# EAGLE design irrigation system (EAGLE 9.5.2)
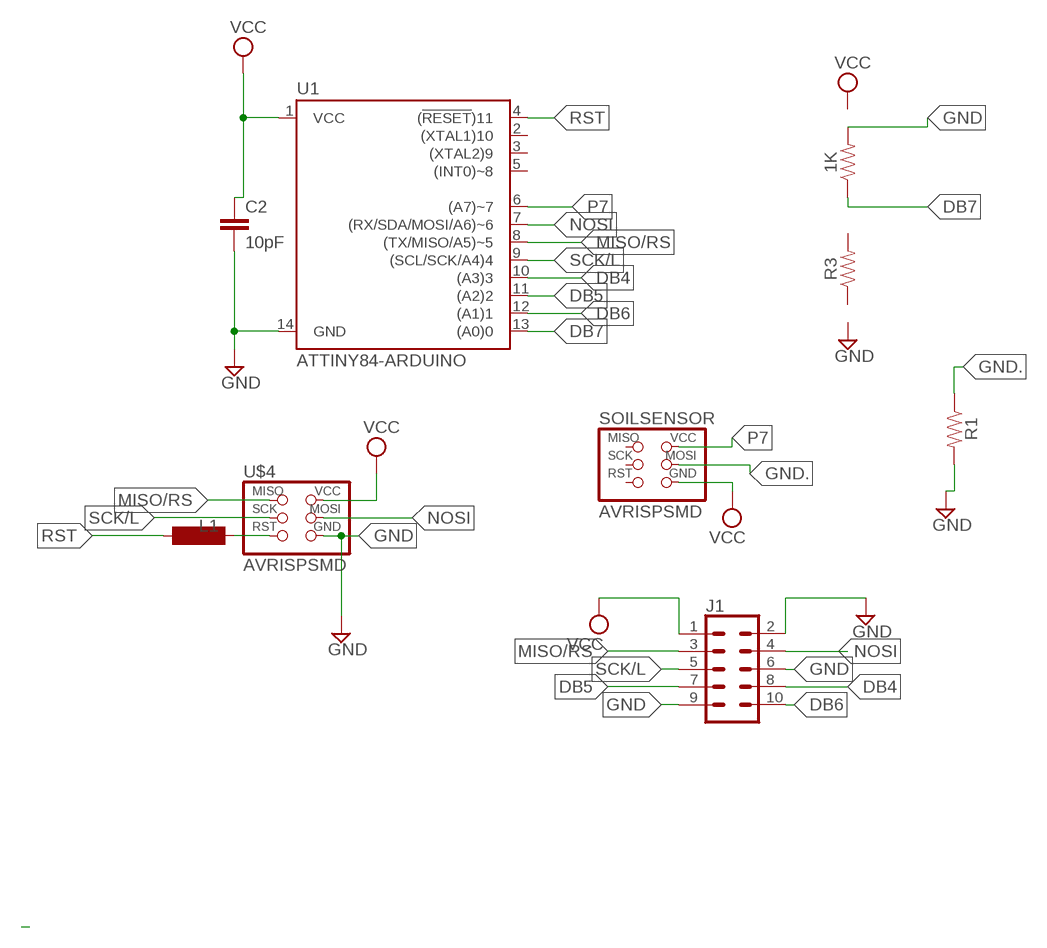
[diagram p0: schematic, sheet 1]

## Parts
1K  RESISTOR1206  [1206]
C2  10pF  10PF-0603-50V-5%  [0603]
J1  CONN_05X2SHD_SMD  [2X5-SHROUDED_SMD]
L1  SM-1206  [SM-1206]
R1  RESISTOR1206  [1206]
R3  RESISTOR1206  [1206]
SOILSENSOR  AVRISPSMD  [2X03SMD]
U1  ATTINY84-ARDUINO  [SO14]
U$4  AVRISPSMD  [2X03SMD]

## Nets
DB4: J1.8 U1.10((A3)3)
DB5: J1.7 U1.11((A2)2)
DB6: J1.10 U1.12((A1)1)
DB7: 1K.1 U1.13((A0)0)
GND: 1K.2 C2.2 J1.2 J1.6 J1.9 R1.2 U1.14(GND) U$4.6(GND)
GND.: R1.1 SOILSENSOR.4(MOSI)
MISO/RS: J1.3 U1.8((TX/MISO/A5)~5) U$4.1(MISO)
N$6: L1.2 U$4.5(RST)
NOSI: J1.4 U1.7((RX/SDA/MOSI/A6)~6) U$4.4(MOSI)
P7: SOILSENSOR.2(VCC) U1.6((A7)~7)
RST: L1.1 U1.4((!RESET!)11)
SCK/L: J1.5 U1.9((SCL/SCK/A4)4) U$4.3(SCK)
VCC: C2.1 J1.1 SOILSENSOR.6(GND) U1.1(VCC) U$4.2(VCC)
Unconnected: R3.1 R3.2 SOILSENSOR.1(MISO) SOILSENSOR.3(SCK) SOILSENSOR.5(RST) U1.2((XTAL1)10) U1.3((XTAL2)9) U1.5((INT0)~8)

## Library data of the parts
1K R1 R3 = SparkFun-Resistors:RESISTOR: Generic Resistor Package
C2 = SparkFun-Capacitors:10PF: 10pF ceramic capacitors; PROD_ID: CAP-11812
J1 = SparkFun-Connectors:CONN_05X2: Multi connection point. Often used as Generic Header-pin footprint for 0.1 inch spaced/style header connections For AVR SPI programming port, see special device with nice symbol: "AVR_SPI_PROG_5x2.dev" You can populate with any combo of single row headers, but if you'd like an exact match, check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; PROD_ID: CONN-09508
L1 = inductor-neosid:SM-1206: INDUCTOR; OC_FARNELL: unknown; OC_NEWARK: unknown
SOILSENSOR U$4 = fab:AVRISP
U1 = SparkFun-IC-Microcontroller:ATTINY84-ARDUINO; PROD_ID: IC-14155

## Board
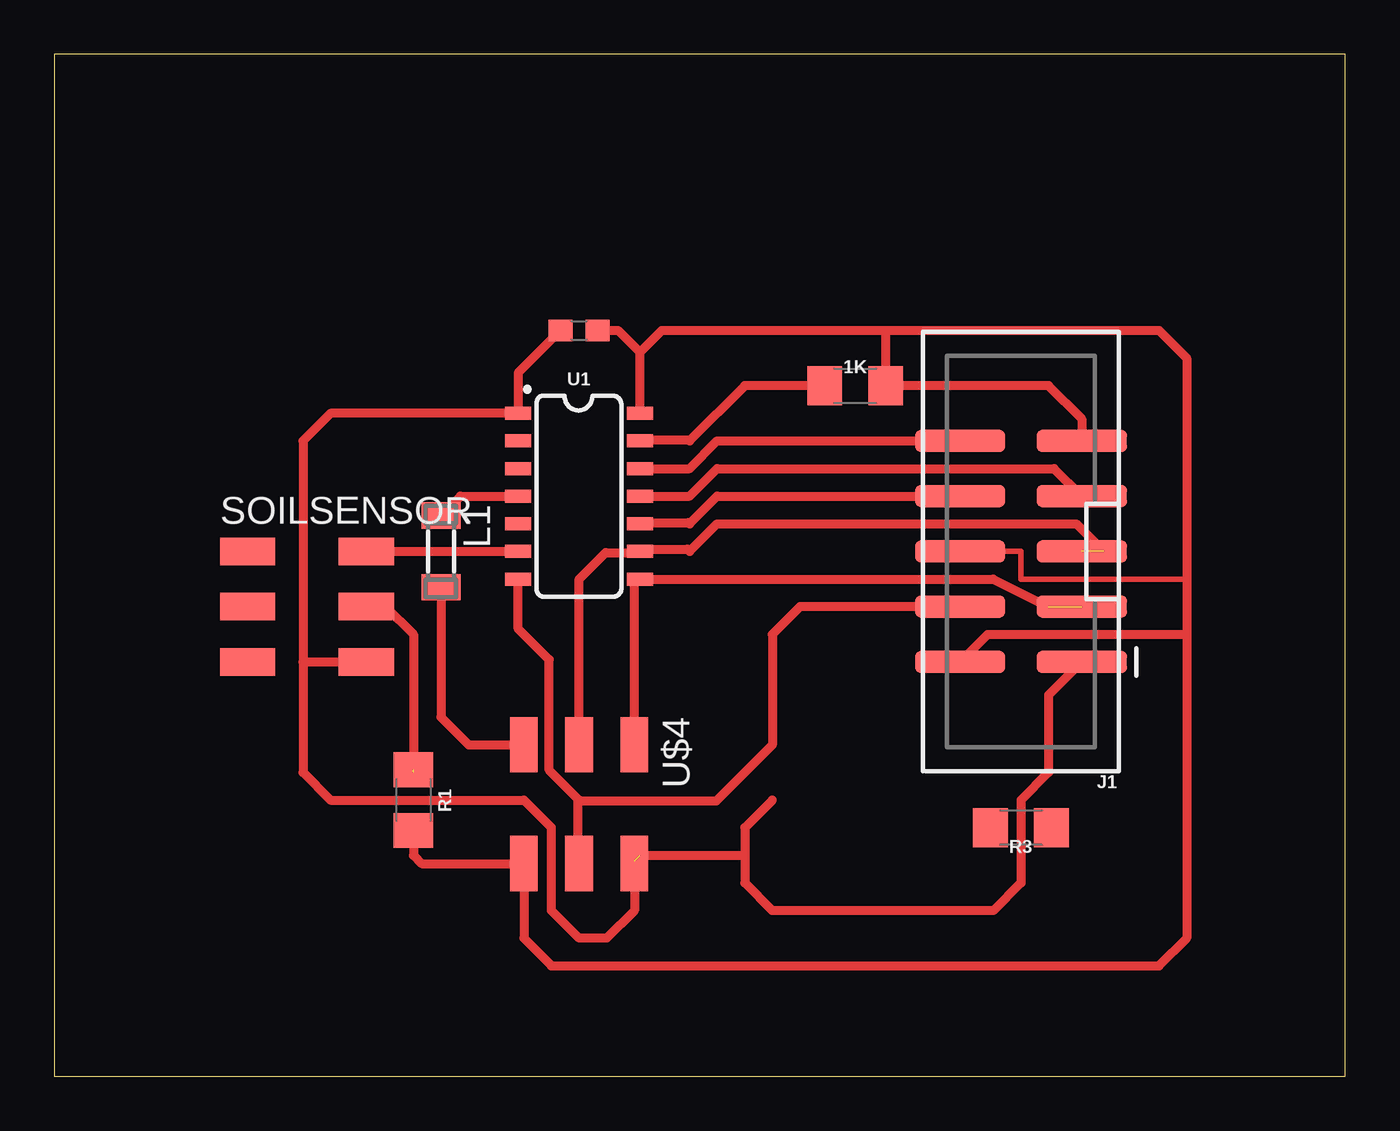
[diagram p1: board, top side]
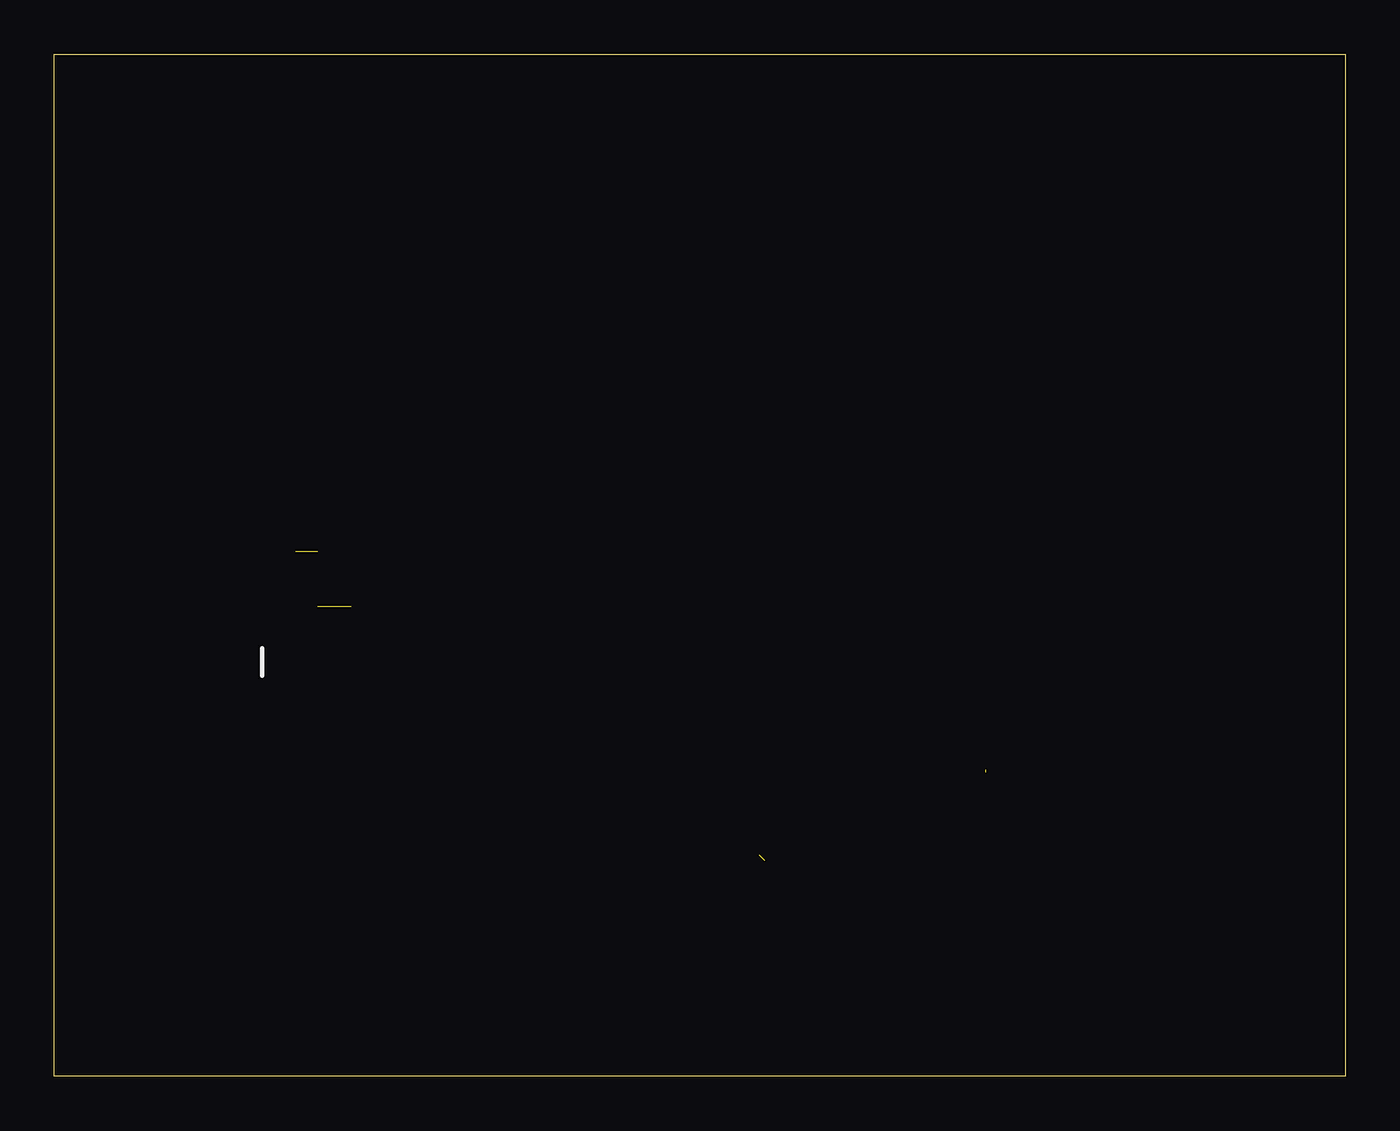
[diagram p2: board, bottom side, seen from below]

Size 59.36 x 46.98 mm. Coordinates in mm from the lower left corner, seen from the top.
Outline: 0,0 59.36,0 59.36,46.98 0,46.98 0,0
Copper layers (1*16): Top 0.035mm / dielectric 1.5mm / Bottom 0.035mm
Design rules "default": minimum track width 6mil, minimum drill 0.35mm, track to track 6mil, track to pad 6mil, pad to pad 6mil, via to via 6mil, smd to smd 6mil, copper to edge 40mil, drill to drill 6mil, minimum pad ring 10mil, minimum via ring 8mil, stop-mask expansion 4mil, vias tented up to drill 0mil, thermal gap 10mil

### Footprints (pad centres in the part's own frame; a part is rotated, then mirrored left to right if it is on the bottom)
1206 = smd 1.6 x 1.8: 1 -1.4,0; 2 1.4,0
0603 = smd 1.1 x 1: 1 -0.85,0; 2 0.85,0
2X5-SHROUDED_SMD = smd 4.15 x 1: 1 -2.794,5.08; 2 2.794,5.08; 3 -2.794,2.54; 4 2.794,2.54; 5 -2.794,0; 6 2.794,0; 7 -2.794,-2.54; 8 2.794,-2.54; 9 -2.794,-5.08; 10 2.794,-5.08
SM-1206 = smd 1.2 x 1.8: 1 -1.65,0; 2 1.65,0
2X03SMD = smd 2.54 x 1.27: 1 -2.54,2.54; 2 2.92,2.54; 3 -2.54,0; 4 2.92,0; 5 -2.54,-2.54; 6 2.92,-2.54
SO14 = smd 0.6 x 1.2: 1 -3.81,-2.8; 2 -2.54,-2.8; 3 -1.27,-2.8; 4 0,-2.8; 5 1.27,-2.8; 6 2.54,-2.8; 7 3.81,-2.8; 8 3.81,2.8; 9 2.54,2.8; 10 1.27,2.8; 11 0,2.8; 12 -1.27,2.8; 13 -2.54,2.8; 14 -3.81,2.8

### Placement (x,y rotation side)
1K  36.83,31.75 0 top
C2  24.13,34.29 0 top
J1  44.45,24.13 180 top
L1  17.78,24.13 270 top
R1  16.51,12.7 270 top
R3  44.45,11.43 180 top
SOILSENSOR  11.43,21.59 0 top
U1  24.13,26.67 270 top
U$4  24.13,12.7 270 top

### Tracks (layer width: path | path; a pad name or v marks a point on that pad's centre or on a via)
DB4
  Top 0.152: 26.98,25.3 U1.10 26.98,25.45 | 29.16,25.45 29.21,25.4
  Top 0.406: 26.98,25.45 29.16,25.45 | 29.21,25.4 30.48,26.67 J1.8
DB5
  Top 0.406: U1.11 29.21,26.67 30.48,27.94 45.97,27.94 J1.7
DB6
  Top 0.152: U1.12 26.98,28.04
  Top 0.406: J1.10 30.48,29.21 29.21,27.94 U1.12
DB7
  Top 0.152: U1.13 26.98,29.26 | 29.21,29.21 29.16,29.26
  Top 0.406: 26.98,29.26 29.16,29.26 | 1K.1 31.75,31.75 29.21,29.21
GND
  Top 0.152: C2.2 24.84,34.29 | U1.14 26.52,30.48 | U$4.6 21.64,9.75 | 41.76,24.13 J1.6
  Top 0.254: J1.6 44.45,24.13 44.45,22.86 52.07,22.86
  Top 0.406: U1.14 26.93,33.28 | 26.93,33.28 27.94,34.29 38.1,34.29 | 38.1,34.29 50.8,34.29 52.07,33.02 52.07,22.86 52.07,20.32 | 52.07,20.32 52.07,6.35 50.8,5.08 22.86,5.08 21.59,6.35 U$4.6 16.89,9.78 16.51,10.16 R1.2 | C2.2 25.92,34.29 26.93,33.28 | J1.2 42.93,20.32 52.07,20.32 | J1.9 47.24,30.23 45.72,31.75 1K.2 38.23,34.16 38.1,34.29
GND.  (1 unrouted)
  Top 0.406: SOILSENSOR.4 15.24,21.59 16.51,20.32 16.51,13.97
MISO/RS  (1 unrouted)
  Top 0.152: 47.24,21.54 J1.3 | 26.67,22.86 U1.8
  Top 0.406: U$4.1 26.67,22.86 | U1.8 43.18,22.86 45.72,21.59
N$6
  Top 0.152: 17.88,22.4 L1.2 | 21.49,15.24 U$4.5
  Top 0.406: L1.2 17.78,16.51 19.05,15.24 U$4.5
NOSI
  Top 0.152: U1.7 | U$4.4 24.08,9.91 | 24.08,12.65 24.13,12.7
  Top 0.406: 24.08,9.91 24.08,12.65 30.43,12.65 33.02,15.24 33.02,20.32 34.29,21.59 J1.4 | 24.13,12.7 22.76,14.07 22.76,19.15 21.34,20.57 U1.7
P7
  Top 0.406: SOILSENSOR.2 U1.6
RST
  Top 0.152: 17.88,25.91 L1.1
  Top 0.406: L1.1 18.67,26.67 U1.4
SCK/L  (1 unrouted)
  Top 0.152: 26.98,24.08 U1.9 26.98,24.23 | 24.23,15.24 U$4.3 | 29.11,24.23 29.21,24.13
  Top 0.406: U$4.3 24.13,22.86 25.35,24.08 26.98,24.08 | 26.98,24.23 29.11,24.23 | 29.21,24.13 30.48,25.4 46.99,25.4 48.26,24.13
VCC  (1 unrouted)
  Top 0.152: 23.16,34.29 C2.1 23.32,34.29 | U1.1 | U$4.2 26.67,9.91
  Top 0.406: U$4.2 26.67,7.62 25.4,6.35 24.13,6.35 22.86,7.62 22.86,11.43 21.59,12.7 12.7,12.7 11.43,13.97 11.43,19.05 | J1.1 45.72,17.53 45.72,13.97 44.45,12.7 44.45,8.89 43.18,7.62 33.02,7.62 31.75,8.89 31.75,10.16 | C2.1 21.33,32.34 U1.1 12.7,30.48 11.43,29.21 11.43,19.05 | 33.02,12.7 31.75,11.43 31.75,10.16 | 26.92,10.16 31.75,10.16 | 11.43,19.05 SOILSENSOR.6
